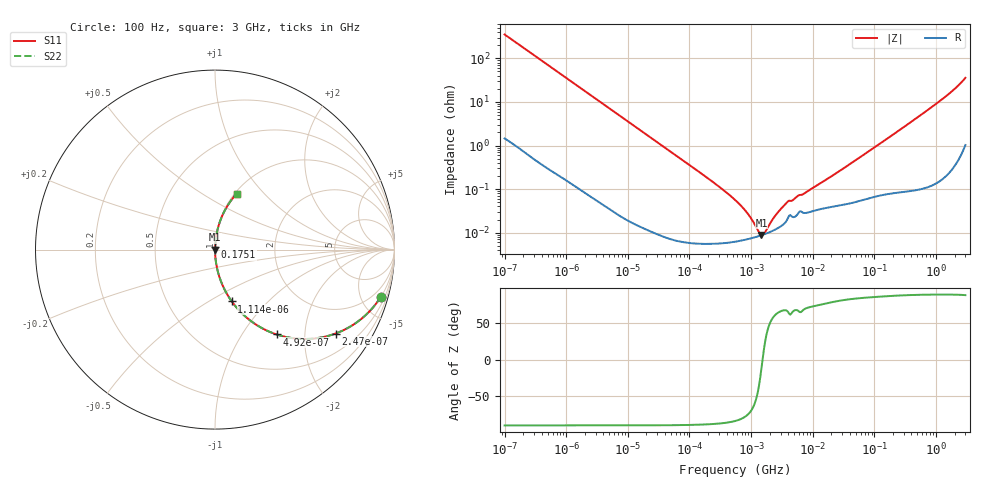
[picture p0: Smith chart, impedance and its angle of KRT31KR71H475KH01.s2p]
!Murata Part Number: KRT31KR71H475KH01
!These Parameters are Measured in Series Mode Connection
!Data Generated on Jan 08, 2026
!  o--ll--o
!Port1  Port2
!  o------o
!Operation Temp=25[degC], DC Bias Voltage=0[V]
!Freq. Start=100[Hz] Stop=3[GHz] 401[Steps]
# Hz S RI R 50
!Freq.(Hz) S11(Real) S11(Imag) S21(Real) S21(Imag) S12(Real) S12(Imag) S22(Real) S22(Imag)
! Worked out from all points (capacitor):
!   401 points, 100 Hz to 3 GHz, reference 50 ohm
!   read as one part in series: C = 4.51 uF near 109 Hz
!   lowest |Z| = 8.92 mohm at 1.474 MHz (marker M1)
!   series resonance near 1.533 MHz, so ESL is about 2.4 nH
!   S11 on the Smith chart (normalised r, x): 100 Hz: 1.03, -7.06; 247 Hz: 1.01, -2.87; 492 Hz: 1.01, -1.44; 1.114 kHz: 1.00, -0.64; 175.1 MHz: 1.00, +0.03; 3 GHz: 1.02, +0.72
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100  0.9248 -0.2617  0.0752 0.2617  0.0752 0.2617  0.9248 -0.2617
161  0.8279 -0.3754  0.1721 0.3754  0.1721 0.3754  0.8279 -0.3754
247  0.6719 -0.4675  0.3281 0.4675  0.3281 0.4675  0.6719 -0.4675
492  0.3427 -0.4725  0.6573 0.4725  0.6573 0.4725  0.3427 -0.4725
724  0.1946 -0.3937  0.8054 0.3937  0.8054 0.3937  0.1946 -0.3937
1114  0.0934 -0.2888  0.9066 0.2888  0.9066 0.2888  0.0934 -0.2888
1788  0.0389 -0.191  0.9611 0.191  0.9611 0.191  0.0389 -0.191
5716  0.00419 -0.0622  0.9958 0.0622  0.9958 0.0622  0.00419 -0.0622
31977  0.000214 -0.0112  0.9998 0.0112  0.9998 0.0112  0.000214 -0.0112
231582  5.78e-05 -0.00151  0.9999 0.00151  0.9999 0.00151  5.78e-05 -0.00151
547723  6.23e-05 -0.000564  0.9999 0.000564  0.9999 0.000564  6.23e-05 -0.000564
842342  7.01e-05 -0.00029  0.9999 0.00029  0.9999 0.00029  7.01e-05 -0.00029
1295438  8.25e-05 -7.6e-05  0.9999 7.6e-05  0.9999 7.6e-05  8.25e-05 -7.6e-05
1473992  8.75e-05 -1.74e-05  0.9999 1.74e-05  0.9999 1.74e-05  8.75e-05 -1.74e-05
1750920  9.54e-05 5.94e-05  0.9999 -5.94e-05  0.9999 -5.94e-05  9.54e-05 5.94e-05
2470636  0.000118 0.000217  0.9999 -0.000217  0.9999 -0.000217  0.000118 0.000217
3799590  0.000193 0.000455  0.9998 -0.000455  0.9998 -0.000455  0.000193 0.000455
9794414  0.00031 0.000997  0.9997 -0.000997  0.9997 -0.000997  0.00031 0.000997
1.751444e8  0.00102 0.0155  0.999 -0.0155  0.999 -0.0155  0.00102 0.0155
1.06781e9  0.0106 0.0955  0.9894 -0.0955  0.9894 -0.0955  0.0106 0.0955
1.868531e9  0.0347 0.175  0.9653 -0.175  0.9653 -0.175  0.0347 0.175
3e9  0.1206 0.3116  0.8794 -0.3116  0.8794 -0.3116  0.1206 0.3116
